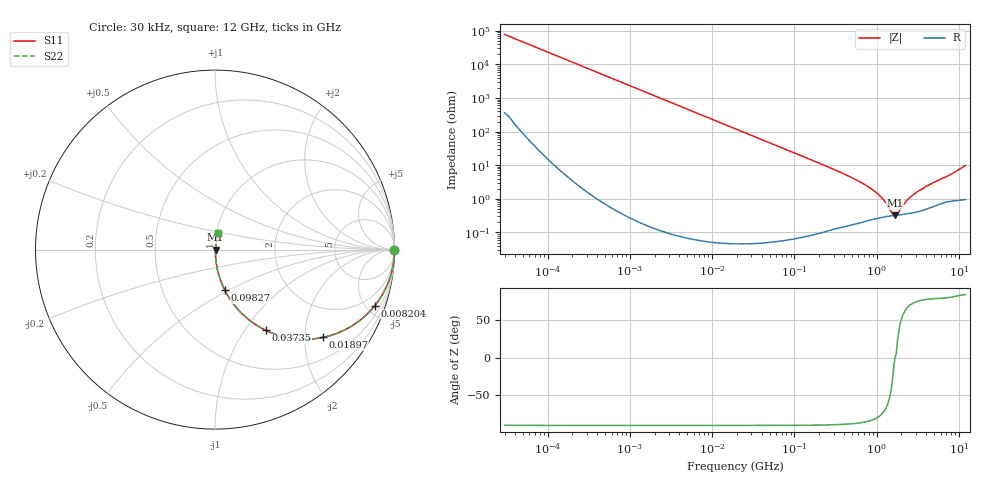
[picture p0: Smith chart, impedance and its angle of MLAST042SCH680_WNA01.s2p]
! MLAST042SCH680_WNA01  S-PARAMETER MODEL  ( General Type )
! Model Generated by TAIYO YUDEN Corporation (http://www.ty-top.com)
! Version 1.0
! TAIYO YUDEN Control No. 150820
! Copyright(c) 2015 TAIYO YUDEN CO.,LTD. All Rights Reserved.
! Product Description (link to TY-COMPAS)
! https://ds.yuden.co.jp/TYCOMPAS/or/detail?pn=MLAST042SCH680JWNA01&u=M
! Products Name : Multilayer Ceramic Capacitors
! Characteristics :
!  Capacitance : 68 pF , Rated Voltage : 25V , TCC : CH / C0H
!  Case Size : 0.4 x 0.2 / 0.016 x 0.008 [mm/inch] , Thickness : 0.2 / 0.008 [mm/inch]
!  (Conditions: Temperature = 25 degC , DC Bias Current/Voltage = 0A / 0V)
! External Node Assignments :
!  1  o---| |---o  2
! GND o---------o GND
! Frequency Range : 0.03MHz  -  12000MHz  [ 401 STEP ]
# MHz S RI R 50
! Freq[MHz].  S11 Real  S11 Imag  S21 Real  S21 Imag  S12 Real  S12 Imag  S22 Real  S22 Imag
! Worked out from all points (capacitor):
!   401 points, 30 kHz to 12 GHz, reference 50 ohm
!   read as one part in series: C = 68 pF near 32 kHz
!   lowest |Z| = 320 mohm at 1.678 GHz (marker M1)
!   series resonance near 1.673 GHz, so ESL is about 130 pH
!   S11 on the Smith chart (normalised r, x): 30 kHz: open; 8.204 MHz: 1.00, -5.71; 18.97 MHz: 1.00, -2.47; 37.35 MHz: 1.00, -1.25; 98.27 MHz: 1.00, -0.47; 12 GHz: 1.02, +0.20
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0.03  1 -0.00128  7.61e-06 0.00128  7.61e-06 0.00128  1 -0.00128
0.260295  0.9999 -0.0111  0.000126 0.0111  0.000126 0.0111  0.9999 -0.0111
2.258455  0.9908 -0.0956  0.00924 0.0956  0.00924 0.0956  0.9908 -0.0956
4.741653  0.9605 -0.1946  0.0395 0.1946  0.0395 0.1946  0.9605 -0.1946
8.203843  0.8905 -0.3121  0.1095 0.3121  0.1095 0.3121  0.8905 -0.3121
12.47626  0.7786 -0.415  0.2214 0.415  0.2214 0.415  0.7786 -0.415
18.97367  0.6033 -0.489  0.3967 0.489  0.3967 0.489  0.6033 -0.489
26.19406  0.4439 -0.4966  0.5561 0.4966  0.5561 0.4966  0.4439 -0.4966
37.34732  0.2819 -0.4496  0.7181 0.4496  0.7181 0.4496  0.2819 -0.4496
58.65857  0.1374 -0.3436  0.8626 0.3436  0.8626 0.3436  0.1374 -0.3436
98.2684  0.0539 -0.2244  0.9461 0.2244  0.9461 0.2244  0.0539 -0.2244
164.6252  0.0202 -0.1378  0.9798 0.1378  0.9798 0.1378  0.0202 -0.1378
433.1624  0.00404 -0.0501  0.996 0.0501  0.996 0.0501  0.00404 -0.0501
774.0045  0.00277 -0.0235  0.9972 0.0235  0.9972 0.0235  0.00277 -0.0235
1103.571  0.00286 -0.0117  0.9971 0.0117  0.9971 0.0117  0.00286 -0.0117
1428.372  0.00307 -0.00419  0.9969 0.00419  0.9969 0.00419  0.00307 -0.00419
1573.464  0.00315 -0.00145  0.9969 0.00145  0.9969 0.00145  0.00315 -0.00145
1678.29  0.00319 5.75e-05  0.9968 -5.75e-05  0.9968 -5.75e-05  0.00319 5.75e-05
1790.1  0.00324 0.00135  0.9968 -0.00135  0.9968 -0.00135  0.00324 0.00135
2392.896  0.00366 0.0087  0.9963 -0.0087  0.9963 -0.0087  0.00366 0.0087
3097.169  0.00427 0.0154  0.9957 -0.0154  0.9957 -0.0154  0.00427 0.0154
12000  0.0186 0.0949  0.9814 -0.0949  0.9814 -0.0949  0.0186 0.0949
